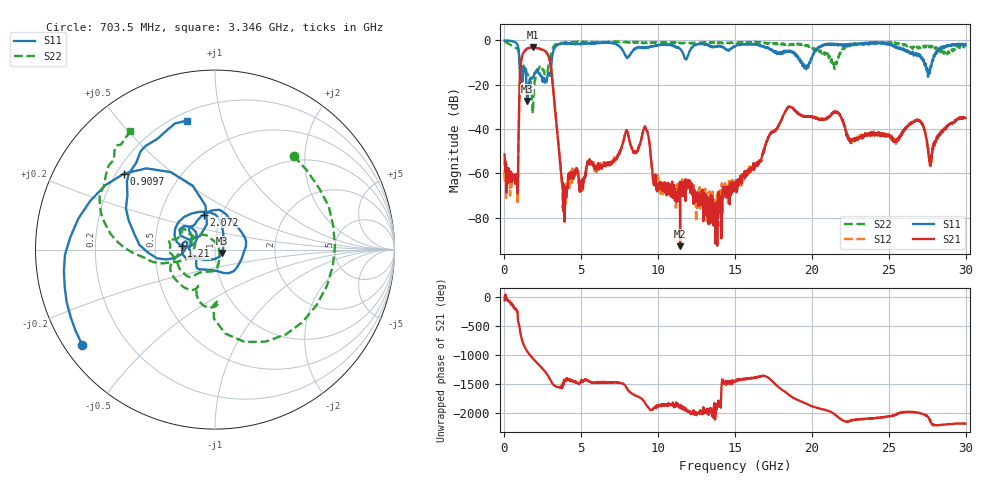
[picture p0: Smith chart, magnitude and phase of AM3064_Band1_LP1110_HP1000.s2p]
# Hz S DB R 50.0
!freq dBS11 angS11 dBS21 angS21 dBS12 angS12 dBS22 angS22
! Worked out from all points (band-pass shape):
!   1600 points, 10 MHz to 29.98 GHz, reference 50 ohm
!   highest |S21| = -3.18 dB at 1.828 GHz (marker M1); lowest = -92.8 dB at 11.42 GHz (marker M2)
!   |S21| within 3 dB of the highest: 1.188 GHz to 2.803 GHz (1.615 GHz wide, 80.9 % of centre)
!   lowest |S11| = -27.3 dB at 1.491 GHz (marker M3), VSWR 1.09, Z = 54 - j2.01 ohm
!   |S11| at or under -10 dB: 974 MHz to 3.062 GHz (2.087 GHz wide, 103 % of centre); 19.36 GHz to 19.82 GHz (464.5 MHz wide, 2.37 % of centre); 27.3 GHz to 27.8 GHz (495.7 MHz wide, 1.8 % of centre)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
!   |S22| runs from -33.0 to -0.4 dB; largest |S21 - S12| = 0.012
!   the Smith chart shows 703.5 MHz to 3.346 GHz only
!   S11 on the Smith chart (normalised r, x): 703.5 MHz: 0.05, -0.32; 909.7 MHz: 0.23, +0.35; 1.21 GHz: 0.69, +0.03; 2.072 GHz: 0.82, +0.33; 3.346 GHz: 0.25, +0.78
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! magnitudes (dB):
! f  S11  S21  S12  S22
! 10 MHz  0.0  -51.4  -58.3  -0.4
! 703.5 MHz  -0.8  -63.3  -64.0  -3.3
! 909.7 MHz  -3.6  -47.3  -47.4  -4.7
! 1.21 GHz  -14.6  -5.9  -5.8  -12.3
! 1.491 GHz  -27.3  -3.7  -3.6  -15.1
! 1.828 GHz  -16.9  -3.2  -3.2  -32.3
! 2.072 GHz  -13.8  -3.4  -3.4  -14.2
! 2.897 GHz  -14.8  -7.7  -7.6  -10.0
! 3.346 GHz  -2.7  -35.2  -35.2  -1.8
! 3.852 GHz  -1.4  -77.5  -69.8  -1.1
! 5.015 GHz  -1.4  -65.1  -64.7  -0.6
! 9.157 GHz  -3.4  -39.3  -39.2  -1.1
! 10 GHz  -2.2  -67.2  -63.4  -0.9
! 11.42 GHz  -3.8  -92.8  -68.0  -1.3
! 13.71 GHz  -2.9  -73.9  -72.0  -1.2
! 15 GHz  -2.6  -64.0  -65.6  -1.2
! 18.45 GHz  -5.1  -30.2  -30.0  -2.0
! 19.99 GHz  -8.3  -34.3  -34.5  -3.0
! 25 GHz  -1.5  -43.1  -43.1  -1.1
! 26.94 GHz  -6.4  -36.2  -36.4  -3.4
! 27.71 GHz  -11.5  -56.7  -51.7  -2.5
! 29.98 GHz  -1.7  -35.1  -35.1  -3.0
